(* Logix 5000 AddOnInstructionDefinition export AMCI_5034_PTO_AM_Encoder_Follower; software revision 37.00 *)

TYPE AMCI_5034_PTO_AM_Input_Data :
STRUCT
   ConnectionFaulted : DINT;
   MovingCW : BOOL;
   MovingCCW : BOOL;
   InHoldState : BOOL;
   Stopped : BOOL;
   AtHome : BOOL;
   Accelerating : BOOL;
   Decelerating : BOOL;
   MoveComplete : BOOL;
   HomeInvalid : BOOL;
   InvalidProfile : BOOL;
   PositionInvalid : BOOL;
   InputError : BOOL;
   CommandError : BOOL;
   ConfigurationError : BOOL;
   ModuleOK : BOOL;
   GeneralPurposeOutputStatus : BOOL;
   Input1Active : BOOL;
   Input2Active : BOOL;
   Input3Active : BOOL;
   Input4Active : BOOL;
   bit_20_reserved : BOOL;
   bit_21_reserved : BOOL;
   bit_22_reserved : BOOL;
   EncoderFollowerMode : BOOL;
   BlendMoveRunning : BOOL;
   BlendMoveAcknowledge : BOOL;
   MinimumRegistrationProgrammed : BOOL;
   EncoderMotionDirection : BOOL;
   MultipleInputsWithSameFunction : BOOL;
   FSCExceedsNumberOfDataBits : BOOL;
   AbsoluteEncoderSetupError : BOOL;
   bit_31_reserved : BOOL;
   CurrentPosition : DINT;
   EncoderPosition : DINT;
   CapturedPosition : DINT;
END_STRUCT
END_TYPE

TYPE AMCI_5034_PTO_AM_Output_Data :
STRUCT
   Command_Word : DINT;
   TargetPosition : DINT;
   TargetVelocity : UDINT;
   Acceleration : DINT;
   Deceleration : DINT;
END_STRUCT
END_TYPE

ADD_ON_INSTRUCTION AMCI_5034_PTO_AM_Encoder_Follower   (* revision 1.0, vendor AMCI, ExecuteEnableInFalse *)
// AMCI Encoder Follower
// Revision note:
// 10/01/2025  Initial release of AOI.
// Help:
// AXIS INPUT DATA:  Input data from the AMCI 5034-PTO-AM.   Uses the AMCI_5034_PTO_Input_Data User Defined Data Type.
// AXIS OUTPUT DATA; Output data from the AOI to the AMCI 5034-PTO-AM.    Uses the AMCI_5034_PTO_Output_Data User Defined Data Type.
// DIRECTION_0_POSITIVECW_1_NEGATIVECCW: 0 to have the output steps be in the same direction as the encoder pulses.   1 to have the output steps be in the opposite direction from the encoder pulses.
// MULTIPLIER: The incoming encoder data is muliplied by this number.
// DIVISOR: The incomming encoder data is divided by this number.
// ACCELERATION: Acceleration Rate in units of steps / sec / ms.  Can be zero with the encoder follower.
// DECELERATION:  Deceleration Rate in units of steps / sec / ms.  Can be zero with the encoder follower.
// EN (Enable) Set when rung is true, Reset when rung is false
// DN (Done) Set when command is sent to the motion device.  Reset when the rung is false.
// ER (Error) Set when a command or input error failed to clear.  Reset when the rung is false.
// IP (In Process) Set when motion is occurring.   Reset when motion stops or the rung goes false.
VAR_IN_OUT
   Axis_Input_Data : AMCI_5034_PTO_AM_Input_Data; {required}
   Axis_Output_Data : AMCI_5034_PTO_AM_Output_Data; {required}
END_VAR
VAR_INPUT
   Direction_0_PositiveCW_1_NegativeCCW : BOOL; {required}
   Multiplier : DINT; {required}
   Divisor : DINT; {required}
   Acceleration : DINT; {required}
   Deceleration : DINT; {required}
END_VAR
VAR_OUTPUT
   EN : BOOL; {visible}   // set when rung with AOI is true
   DN : BOOL; {access Read Only, visible}   // set when move was succesfully initiated
   ER : BOOL; {visible}
   IP : BOOL; {visible}   // set when motion occurring
END_VAR
VAR
   command_data_block : DINT[5];
        [0]   // Command Word
        [1]   // Target Positon
        [2]   // Programmed Speed
        [3]   // Acceleration
        [4]   // Deceleration
   motion_occurring : BOOL; {access None}
   Internal_Enable : BOOL; {access None}   // set when driver ready to receive motion command
END_VAR

ROUTINE EnableInFalse   (* ladder *)
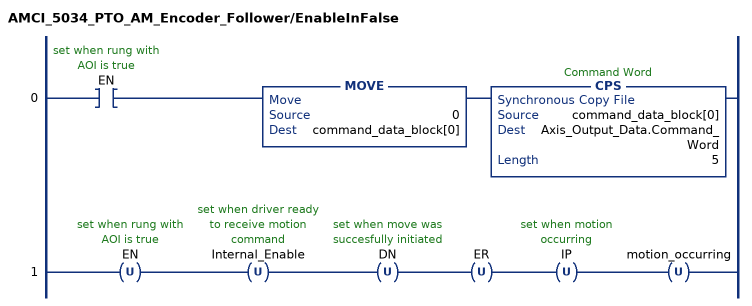
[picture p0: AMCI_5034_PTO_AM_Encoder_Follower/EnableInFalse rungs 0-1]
   0: XIC(EN)MOVE(0,command_data_block[0])CPS(command_data_block[0],Axis_Output_Data.Command_Word,5);
   1: OTU(EN)OTU(Internal_Enable)OTU(DN)OTU(ER)OTU(IP)OTU(motion_occurring);
END_ROUTINE

ROUTINE Logic   (* ladder *)
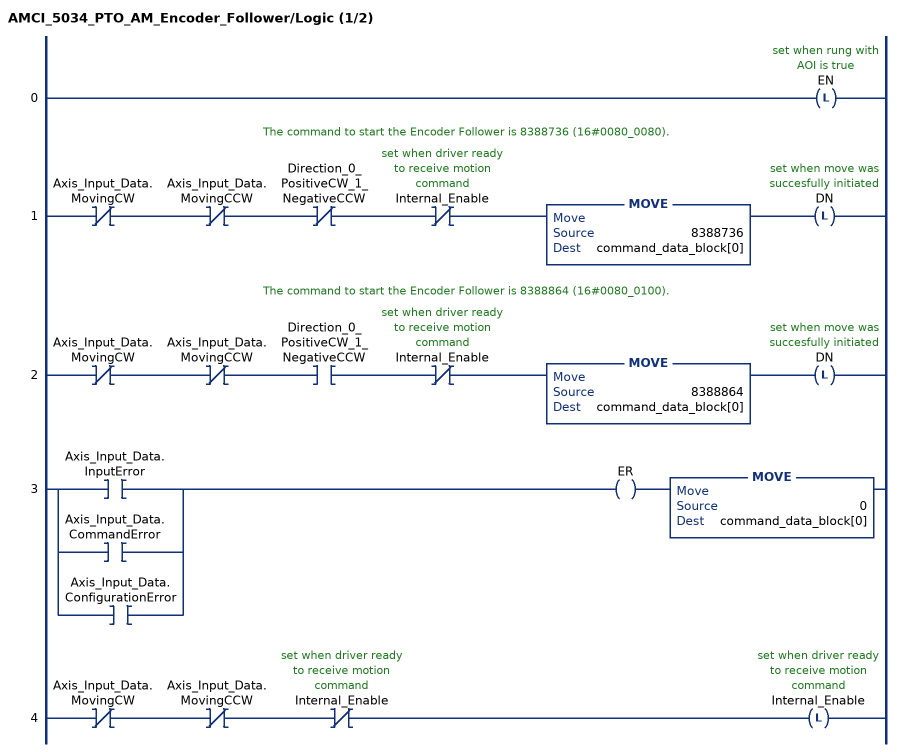
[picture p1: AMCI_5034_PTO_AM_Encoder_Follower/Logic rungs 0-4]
   0: OTL(EN);
   // The command to start the Encoder Follower is 8388736 (16#0080_0080).
   1: XIO(Axis_Input_Data.MovingCW)XIO(Axis_Input_Data.MovingCCW)XIO(Direction_0_PositiveCW_1_NegativeCCW)XIO(Internal_Enable)MOVE(8388736,command_data_block[0])OTL(DN);
   // The command to start the Encoder Follower is 8388864 (16#0080_0100).
   2: XIO(Axis_Input_Data.MovingCW)XIO(Axis_Input_Data.MovingCCW)XIC(Direction_0_PositiveCW_1_NegativeCCW)XIO(Internal_Enable)MOVE(8388864,command_data_block[0])OTL(DN);
   3: [XIC(Axis_Input_Data.InputError) ,XIC(Axis_Input_Data.CommandError) ,XIC(Axis_Input_Data.ConfigurationError) ]OTE(ER)MOVE(0,command_data_block[0]);
   4: XIO(Axis_Input_Data.MovingCW)XIO(Axis_Input_Data.MovingCCW)XIO(Internal_Enable)OTL(Internal_Enable);
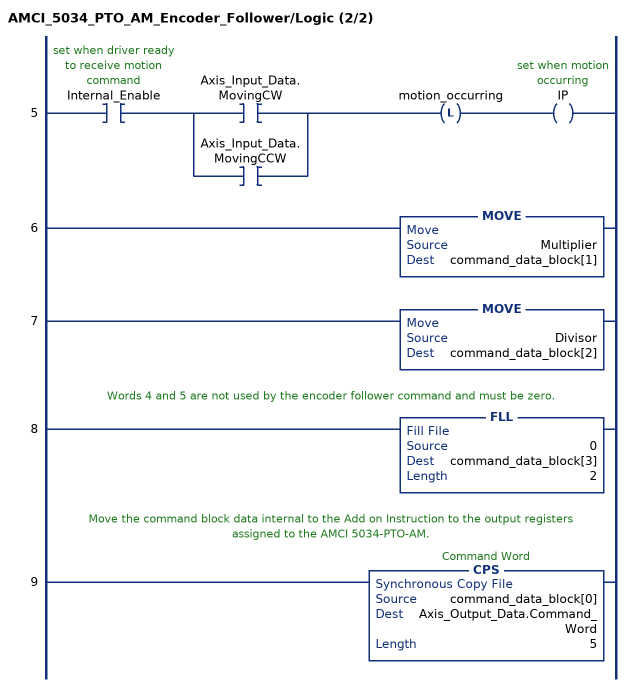
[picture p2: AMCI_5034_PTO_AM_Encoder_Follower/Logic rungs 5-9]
   5: XIC(Internal_Enable)[XIC(Axis_Input_Data.MovingCW) ,XIC(Axis_Input_Data.MovingCCW) ]OTL(motion_occurring)OTE(IP);
   6: MOVE(Multiplier,command_data_block[1]);
   7: MOVE(Divisor,command_data_block[2]);
   // Words 4 and 5 are not used by the encoder follower command and must be zero.
   8: FLL(0,command_data_block[3],2);
   // Move the command block data internal to the Add on Instruction to the output registers assigned to the AMCI 5034-PTO-AM.
   9: CPS(command_data_block[0],Axis_Output_Data.Command_Word,5);
END_ROUTINE
END_ADD_ON_INSTRUCTION
